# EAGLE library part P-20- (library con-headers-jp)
HEADER PLUG PINS
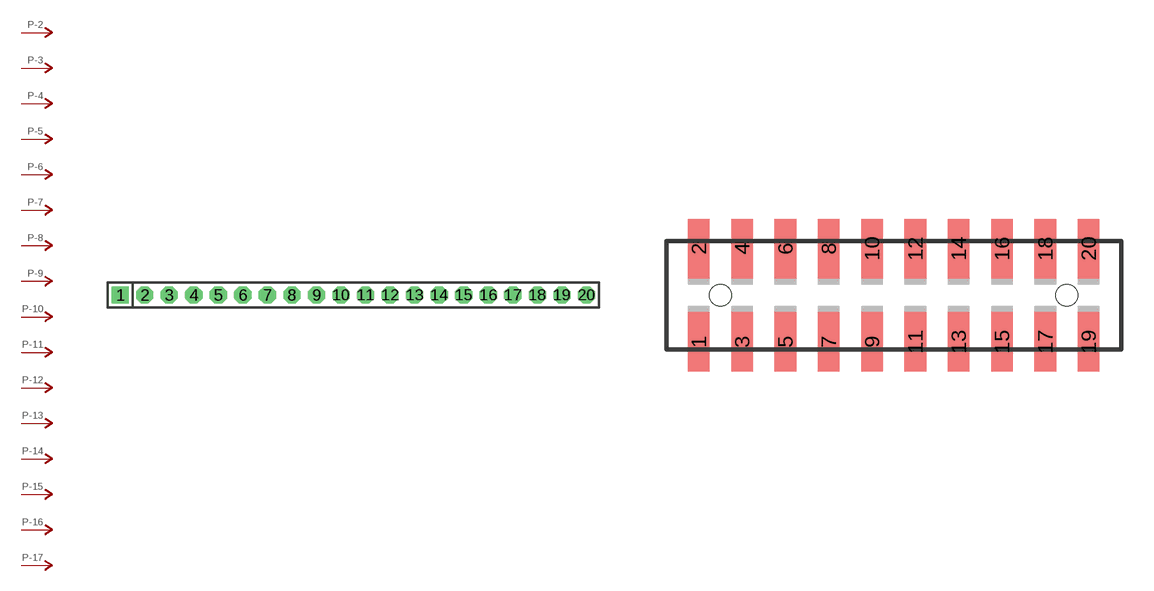
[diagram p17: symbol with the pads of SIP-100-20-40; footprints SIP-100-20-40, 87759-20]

Designator prefix P; gates -2=P-N -3=P-N -4=P-N -5=P-N -6=P-N -7=P-N -8=P-N -9=P-N -10=P-N -11=P-N -12=P-N -13=P-N -14=P-N -15=P-N -16=P-N -17=P-N -18=P-N -19=P-N -20=P-N G$1=P-NV

## P-20-SIP-100-40  [SIP-100-20-40]
1  G$1:P  pas
2  -2:P  pas
3  -3:P  pas
4  -4:P  pas
5  -5:P  pas
6  -6:P  pas
7  -7:P  pas
8  -8:P  pas
9  -9:P  pas
10  -10:P  pas
11  -11:P  pas
12  -12:P  pas
13  -13:P  pas
14  -14:P  pas
15  -15:P  pas
16  -16:P  pas
17  -17:P  pas
18  -18:P  pas
19  -19:P  pas
20  -20:P  pas

## P-20-87759  [87759-20]
Pads as for SIP-100-20-40

## P-20-100-2X10  [DIL-100-2X10]
Pads as for SIP-100-20-40

## P-20-100-2X10_M  [DIL-100-2X10_M]
Pads as for SIP-100-20-40

## P-20-2MM-2X10  [DIL-2MM-2X10]
Pads as for SIP-100-20-40

## P-20-2MM-2X10_M  [DIL-2MM-2X10_M]
Pads as for SIP-100-20-40

## P-20-SIP-100-32  [SIP-100-20-32]
Pads as for SIP-100-20-40

## P-20-SIP-100-40Y  [SIP-100-20-40Y]
Pads as for SIP-100-20-40

## P-20-SIP-100-32Y  [SIP-100-20-32Y]
Pads as for SIP-100-20-40

## P-20-87759_M  [87759-20_M]
Pads as for SIP-100-20-40

## Footprint SIP-100-20-40 (pad centres in mm)
SIP Header - 0.1", 40 mil drill
drill 1.016 pad 1.778 square: 1 -24.13,0
drill 1.016 pad 1.778 octagon: 2 -21.59,0; 3 -19.05,0; 4 -16.51,0; 5 -13.97,0; 6 -11.43,0; 7 -8.89,0; 8 -6.35,0; 9 -3.81,0; 10 -1.27,0; 11 1.27,0; 12 3.81,0; 13 6.35,0; 14 8.89,0; 15 11.43,0; 16 13.97,0; 17 16.51,0; 18 19.05,0; 19 21.59,0; 20 24.13,0

## Footprint 87759-20 (pad centres in mm)
Molex PCB Pin Headers 2.00mm (.079") Pitch Milli-Grid Header, Vertical SMD
smd 1 x 2.75: 1 -9,-2.15; 2 -9,2.15; 3 -7,-2.15; 4 -7,2.15; 5 -5,-2.15; 6 -5,2.15; 7 -3,-2.15; 8 -3,2.15; 9 -1,-2.15; 10 -1,2.15; 11 1,-2.15; 12 1,2.15; 13 3,-2.15; 14 3,2.15; 15 5,-2.15; 16 5,2.15; 17 7,-2.15; 18 7,2.15; 19 9,-2.15; 20 9,2.15
hole 1 at -8,0
hole 1 at 8,0

## Footprint DIL-100-2X10 (pad centres in mm)
PIN HEADER - 0.1"
drill 1.016 square: 1 -11.43,-1.27
drill 1.016 octagon: 2 -11.43,1.27; 3 -8.89,-1.27; 4 -8.89,1.27; 5 -6.35,-1.27; 6 -6.35,1.27; 7 -3.81,-1.27; 8 -3.81,1.27; 9 -1.27,-1.27; 10 -1.27,1.27; 11 1.27,-1.27; 12 1.27,1.27; 13 3.81,-1.27; 14 3.81,1.27; 15 6.35,-1.27; 16 6.35,1.27; 17 8.89,-1.27; 18 8.89,1.27; 19 11.43,-1.27; 20 11.43,1.27

## Footprint DIL-100-2X10_M (pad centres in mm)
PIN HEADER - MIRRORED 0.1"
drill 1.016 square: 1 -11.43,1.27
drill 1.016 octagon: 2 -11.43,-1.27; 3 -8.89,1.27; 4 -8.89,-1.27; 5 -6.35,1.27; 6 -6.35,-1.27; 7 -3.81,1.27; 8 -3.81,-1.27; 9 -1.27,1.27; 10 -1.27,-1.27; 11 1.27,1.27; 12 1.27,-1.27; 13 3.81,1.27; 14 3.81,-1.27; 15 6.35,1.27; 16 6.35,-1.27; 17 8.89,1.27; 18 8.89,-1.27; 19 11.43,1.27; 20 11.43,-1.27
